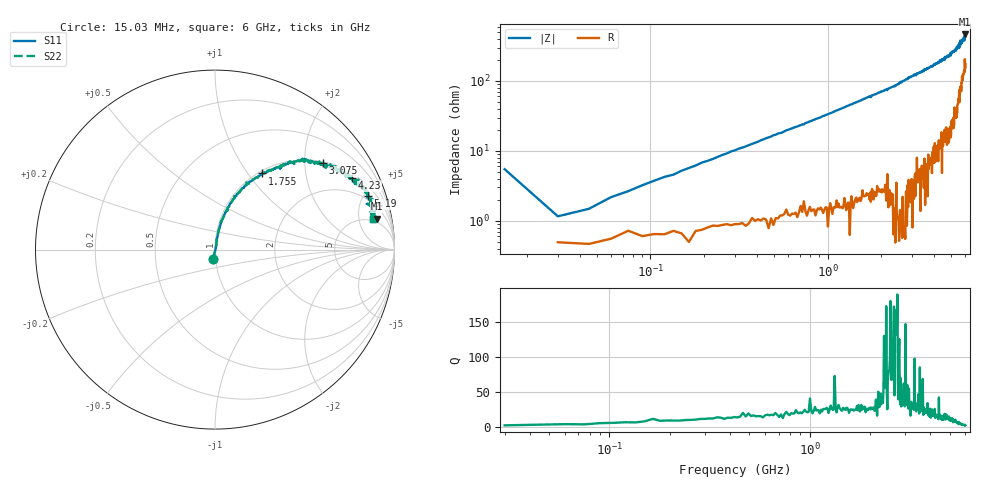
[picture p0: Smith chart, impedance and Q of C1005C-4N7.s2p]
!	Network	Analyzer	HP8753E.07.74:	Oct	30	2002	Serial	No.	JP38451487
!	Hewlett-Packard
!	7	Sep	2009	8:26:39
!	Frequency	S11	S21	S12	S22
#	HZ	S	RI	R	50
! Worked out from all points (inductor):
!   400 points, 15.03 MHz to 6 GHz, reference 50 ohm
!   read as one part in series: L = 5.43 nH near 45.03 MHz
!   highest |Z| = 462 ohm at 5.985 GHz (marker M1)
!   S11 on the Smith chart (normalised r, x): 15.03 MHz: 0.97, -0.11; 1.755 GHz: 1.04, +1.17; 3.075 GHz: 1.04, +2.47; 4.23 GHz: 1.22, +3.71; 5.19 GHz: 1.70, +5.35; 6 GHz: 4.49, +7.98
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1.502992e7  -0.0116 -0.0544  1.01 0.0544  1.01 0.0544  -0.0116 -0.0544
3.002985e7  0.00506 0.0104  0.995 -0.0104  0.995 -0.0104  0.00506 0.0104
6.00297e7  0.00595 0.0209  0.994 -0.0209  0.994 -0.0209  0.00595 0.0209
1.200294e8  0.00823 0.0414  0.992 -0.0414  0.992 -0.0414  0.00823 0.0414
2.850286e8  0.0177 0.0954  0.982 -0.0954  0.982 -0.0954  0.0177 0.0954
5.850271e8  0.0499 0.184  0.95 -0.184  0.95 -0.184  0.0499 0.184
1.020025e9  0.114 0.297  0.886 -0.297  0.886 -0.297  0.114 0.297
1.755021e9  0.262 0.424  0.738 -0.424  0.738 -0.424  0.262 0.424
2.01002e9  0.334 0.452  0.666 -0.452  0.666 -0.452  0.334 0.452
3.015015e9  0.581 0.49  0.419 -0.49  0.419 -0.49  0.581 0.49
3.075015e9  0.603 0.481  0.397 -0.481  0.397 -0.481  0.603 0.481
4.00501e9  0.745 0.417  0.255 -0.417  0.255 -0.417  0.745 0.417
4.230009e9  0.763 0.397  0.237 -0.397  0.237 -0.397  0.763 0.397
5.010005e9  0.84 0.327  0.16 -0.327  0.16 -0.327  0.84 0.327
5.190004e9  0.85 0.298  0.15 -0.298  0.15 -0.298  0.85 0.298
5.535002e9  0.845 0.255  0.155 -0.255  0.155 -0.255  0.845 0.255
5.625002e9  0.893 0.217  0.107 -0.217  0.107 -0.217  0.893 0.217
5.655002e9  0.873 0.235  0.127 -0.235  0.127 -0.235  0.873 0.235
5.865001e9  0.89 0.19  0.11 -0.19  0.11 -0.19  0.89 0.19
5.925e9  0.871 0.197  0.129 -0.197  0.129 -0.197  0.871 0.197
5.985e9  0.901 0.172  0.0992 -0.172  0.0992 -0.172  0.901 0.172
6e9  0.883 0.17  0.117 -0.17  0.117 -0.17  0.883 0.17
